//{attribute 'qualified_only'}
VAR_GLOBAL CONSTANT
	cMinAxis			:	UINT := 1;
	cMaxAxis			:	UINT := 5;
END_VAR         		
VAR_GLOBAL      		
	arAxis				:	ARRAY[cMinAxis..cMaxAxis] OF FB_AxisPtp;
END_VAR
